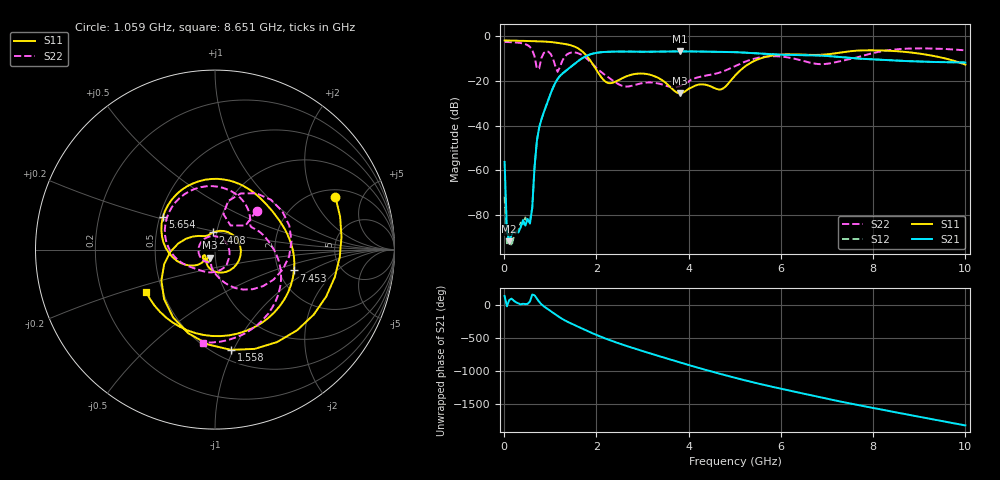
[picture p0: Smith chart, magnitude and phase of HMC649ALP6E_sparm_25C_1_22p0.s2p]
!Analog Devices Inc..
!GaAs MMIC 6-BIT DIGITAL PHASE SHIFTER, 3 - 6 GHz
!Filename: HMC649ALP6E_sparm_25C_1_22p0.s2p
!  :25C = 25degC
!  :_1_ = Sn1
!  :_22p0  = 22.0 state
!Device type:
!2 Port Calibration to sma connectors
!Phase Shifter:  0.000
!	Vss= -5V, Vdd= +5V , control Voltage = 0/ +5V
!Freq	S11	S11	S21	S21	S12	S12	S22	S22
! GHz	Mag dB	Degrees	Mag dB	Degrees	Mag dB	Degrees	Mag dB	Degrees
# GHZ S DB R 50.0
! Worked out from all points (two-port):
!   201 points, 10 MHz to 10 GHz, reference 50 ohm
!   highest |S21| = -6.79 dB at 3.806 GHz (marker M1); lowest = -91.7 dB at 109.9 MHz (marker M2)
!   |S21| within 3 dB of the highest: 1.698 GHz to 7.529 GHz (5.831 GHz wide, 126 % of centre)
!   lowest |S11| = -25.6 dB at 3.806 GHz (marker M3), VSWR 1.11, Z = 47.1 - j4.16 ohm
!   |S11| at or under -10 dB: 1.836 GHz to 5.549 GHz (3.713 GHz wide, 101 % of centre); 9.574 GHz to end of sweep
!   |S22| runs from -22.8 to -2.6 dB; largest |S21 - S12| = 0.0017
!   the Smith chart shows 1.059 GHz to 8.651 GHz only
!   S11 on the Smith chart (normalised r, x): 1.059 GHz: 2.40, +3.02; 1.558 GHz: 0.60, -0.98; 2.408 GHz: 0.96, +0.18; 5.654 GHz: 0.52, +0.21; 7.453 GHz: 2.43, -0.71; 8.651 GHz: 0.40, -0.24
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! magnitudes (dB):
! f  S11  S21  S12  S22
! 10 MHz  -1.9  -56.2  -71.6  -2.6
! 59.95 MHz  -1.9  -86.7  -92.5  -2.6
! 109.9 MHz  -1.9  -91.7  -88.1  -2.6
! 559.5 MHz  -2.2  -83.7  -82.4  -4.8
! 609.4 MHz  -2.2  -76.5  -76.7  -6.2
! 659.4 MHz  -2.2  -58.4  -58.3  -9.0
! 759.2 MHz  -2.3  -40.8  -40.8  -14.4
! 859.1 MHz  -2.4  -34.0  -34.0  -7.5
! 1.059 GHz  -2.7  -23.1  -23.0  -10.0
! 1.159 GHz  -3.0  -19.1  -19.1  -15.9
! 1.558 GHz  -4.9  -11.8  -11.8  -7.4
! 1.708 GHz  -7.1  -9.7  -9.7  -8.7
! 2.408 GHz  -20.4  -6.9  -6.9  -20.5
! 3.357 GHz  -18.8  -6.9  -6.9  -21.2
! 3.806 GHz  -25.6  -6.8  -6.8  -22.3
! 5.005 GHz  -17.6  -7.1  -7.1  -13.4
! 5.654 GHz  -9.3  -7.9  -7.9  -9.2
! 6.703 GHz  -8.4  -8.5  -8.5  -12.1
! 7.453 GHz  -6.8  -9.7  -9.7  -10.5
! 8.352 GHz  -6.5  -10.8  -10.7  -6.2
! 8.651 GHz  -6.9  -11.0  -11.0  -5.6
! 10 GHz  -12.7  -11.8  -11.7  -6.3
